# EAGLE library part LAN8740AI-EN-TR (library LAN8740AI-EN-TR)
Ethernet ICs Small Footprint MII/RMII 10/100 Energy Efficient Ethernet Transceiver Source: Datasheet
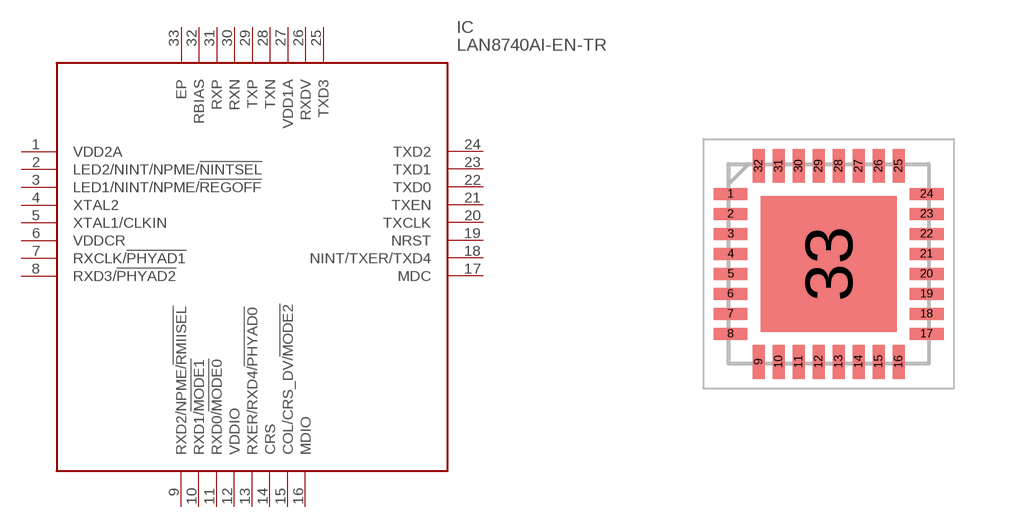
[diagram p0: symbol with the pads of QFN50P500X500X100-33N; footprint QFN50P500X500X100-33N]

Designator prefix IC

## LAN8740AI-EN-TR (Description: Ethernet ICs Small Footprint MII/RMII 10/100 Energy Efficient Ethernet Transceiver; Height: 1mm; Manufacturer_Name: Microchip; Manufacturer_Part_Number: LAN8740AI-EN-TR; Mouser_Part_Number: 579-LAN8740AI-EN-TR; Mouser_Price-Stock: https://www.mouser.co.uk/ProductDetail/Microchip-Technology/LAN8740AI-EN-TR?qs=6qKXPk0vzx1pdBrIaNrUbA%3D%3D)  [QFN50P500X500X100-33N]
1  VDD2A
2  LED2/NINT/NPME/!NINTSEL
3  LED1/NINT/NPME/!REGOFF
4  XTAL2
5  XTAL1/CLKIN
6  VDDCR
7  RXCLK/!PHYAD1
8  RXD3/!PHYAD2
9  RXD2/NPME/!RMIISEL
10  RXD1/!MODE1
11  RXD0/!MODE0
12  VDDIO
13  RXER/RXD4/!PHYAD0
14  CRS
15  COL/CRS_DV/!MODE2
16  MDIO
17  MDC
18  NINT/TXER/TXD4
19  NRST
20  TXCLK
21  TXEN
22  TXD0
23  TXD1
24  TXD2
25  TXD3
26  RXDV
27  VDD1A
28  TXN
29  TXP
30  RXN
31  RXP
32  RBIAS
33  EP

## Footprint QFN50P500X500X100-33N (pad centres in mm)
32-Lead Very Thin Plastic Quad Flat, No Lead Package
smd 0.85 x 0.3: 1 -2.45,1.75; 2 -2.45,1.25; 3 -2.45,0.75; 4 -2.45,0.25; 5 -2.45,-0.25; 6 -2.45,-0.75; 7 -2.45,-1.25; 8 -2.45,-1.75; 17 2.45,-1.75; 18 2.45,-1.25; 19 2.45,-0.75; 20 2.45,-0.25; 21 2.45,0.25; 22 2.45,0.75; 23 2.45,1.25; 24 2.45,1.75
smd 0.3 x 0.85: 9 -1.75,-2.45; 10 -1.25,-2.45; 11 -0.75,-2.45; 12 -0.25,-2.45; 13 0.25,-2.45; 14 0.75,-2.45; 15 1.25,-2.45; 16 1.75,-2.45; 25 1.75,2.45; 26 1.25,2.45; 27 0.75,2.45; 28 0.25,2.45; 29 -0.25,2.45; 30 -0.75,2.45; 31 -1.25,2.45; 32 -1.75,2.45
smd 3.4 x 3.4: 33 0,0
